| TEXAS INSTRUMENTS INCORPORATED
| Standard Linear and Logic Group
| IBIS Model of SN74LVCR162245
| 16-BIT BUS TRANSCEIVER WITH 3-STATE OUTPUTS
| This file contains package information for the following:
|  TSSOP 48-pin (DGG) package as [Component] LVCR162245_DGG
|  jrBGA 48-pin (GQL) package as [Component] LVCR162245_GQL
|  jrBGA 48-pin (ZQL) package as [Component] LVCR162245_ZQL
|  SSOP 48-pin (DL) package as [Component] LVCR162245_DL
| This device can be powered at the following Vccs:
|  2.5 volt Vcc
|  3.3 volt Vcc
| This file provides unique models under the [Model Selector] for each Vcc.
| For operation at a specific Vcc, select the appropriate model after each
| [Model Selector] keyword.
[IBIS Ver]   3.2
[Comment char]  |_char
[File Name]   sn74lvcr162245.ibs
[File Rev]   1.3 | a_die
[Date]   May 16, 2007
[Source]   Data created from TI-SPICE simulations at TI-SLL.
[Notes]   The following is an IBIS list for the SN74LVCR162245.
   Please contact sllibis@ti.com with questions and
   comments concerning SLL IBIS models.
   This IBIS model is created from a BA (back annotated netlist)
   - FILE REV HISTORY
   - 1.1 Release IBIS file on 12/20/04
   - 1.2 Release IBIS file on 5/8/07
   - 1.3 Release IBIS file on 7/20/07, using R_load of 50ohm
   - Non-monotonic data in pullup data due to damping resistor.
[Disclaimer] Property of Texas Instruments Incorporated.  Unauthorized
   reproduction and/or distribution is strictly prohibited.
   This product is protected under copyright law.
   Created  2007, (C) Copyright  2007, Texas Instruments
   Incorporated, All Rights Reserved
   UNLESS THERE IS A SIGNED, WRITTEN AGREEMENT TO THE
   CONTRARY, TEXAS INSTRUMENTS (TI) IS PROVIDING THE IBIS
   MODELS  AND WITHOUT ANY WARRANTY, EXPRESSED OR
   IMPLIED.  TI assumes no liability for:
   1) the accuracy of the IBIS models provided to your
   company;
   2) the proper functioning of these IBIS Models in your
   design or for any resulting applications; or
   3) infringement of patents, copyrights or intellectual
   property rights resulting from your use of these IBIS
   models.
   TI provides IBIS Models as a service to our customers.
   You and your company shall not distribute, sell or give
   these models to anyone else without prior written
   permission from TI.
   TI reserves the right to make changes to our products or
   to discontinue any semiconductor product or service
   without notice, and advises our customers to obtain the
   latest version of relevant information to verify, before
   placing orders, that the information being relied on is
   current.
   Please be aware that your receipt and use of the IBIS
   information provided shall serve as acceptance of these
   terms and conditions.  If you do not accept these terms,
   you should return or destroy the IBIS models and any
   other accompanying information immediately.
| Component SN74LVCR162245_DGG 48-PIN TSSOP
[Component]   SN74LVCR162245_DGG
[Manufacturer]   Texas Instruments, Inc.
[Package]
|   typ   min   max
R_pkg   6.200e-02   5.000e-02   7.800e-02
L_pkg   3.527e-09   3.128e-09   4.255e-09
C_pkg   5.300e-13   4.170e-13   6.850e-13
[Pin]   signal_name   model_name   R_pin   L_pin   C_pin
1   1DIR   LVCR162245_DIR   5.000e-02   4.250e-09   6.710e-13
2   1B1   LVCR162245_IO   5.700e-02   3.956e-09   6.740e-13
3   1B2   LVCR162245_IO   7.100e-02   3.922e-09   6.190e-13
4   GND   GND   7.800e-02   3.841e-09   6.180e-13
5   1B3   LVCR162245_IO   5.600e-02   3.535e-09   5.550e-13
6   1B4   LVCR162245_IO   5.800e-02   3.464e-09   5.030e-13
7   VCC   POWER   6.000e-02   3.362e-09   4.980e-13
8   1B5   LVCR162245_IO   6.100e-02   3.293e-09   4.620e-13
9   1B6   LVCR162245_IO   6.300e-02   3.240e-09   4.550e-13
10   GND   GND   6.300e-02   3.175e-09   4.420e-13
11   1B7   LVCR162245_IO   6.400e-02   3.153e-09   4.290e-13
12   1B8   LVCR162245_IO   6.500e-02   3.128e-09   4.180e-13
13   2B1   LVCR162245_IO   6.500e-02   3.128e-09   4.180e-13
14   2B2   LVCR162245_IO   6.400e-02   3.154e-09   4.290e-13
15   GND   GND   6.300e-02   3.174e-09   4.420e-13
16   2B3   LVCR162245_IO   6.300e-02   3.241e-09   4.550e-13
17   2B4   LVCR162245_IO   6.100e-02   3.293e-09   4.620e-13
18   VCC   POWER   6.000e-02   3.362e-09   4.970e-13
19   2B5   LVCR162245_IO   5.800e-02   3.464e-09   5.030e-13
20   2B6   LVCR162245_IO   5.600e-02   3.537e-09   5.600e-13
21   GND   GND   7.700e-02   3.839e-09   6.260e-13
22   2B7   LVCR162245_IO   7.100e-02   3.917e-09   6.270e-13
23   2B8   LVCR162245_IO   5.800e-02   3.955e-09   6.850e-13
24   2DIR   LVCR162245_DIR   5.200e-02   4.255e-09   6.790e-13
25   2NOE   LVCR162245_NOE   5.100e-02   4.254e-09   6.760e-13
26   2A8   LVCR162245_IO   5.800e-02   3.957e-09   6.790e-13
27   2A7   LVCR162245_IO   7.100e-02   3.920e-09   6.210e-13
28   GND   GND   7.800e-02   3.843e-09   6.220e-13
29   2A6   LVCR162245_IO   5.600e-02   3.539e-09   5.600e-13
30   2A5   LVCR162245_IO   5.800e-02   3.466e-09   5.030e-13
31   VCC   POWER   6.000e-02   3.363e-09   4.970e-13
32   2A4   LVCR162245_IO   6.100e-02   3.294e-09   4.620e-13
33   2A3   LVCR162245_IO   6.300e-02   3.241e-09   4.540e-13
34   GND   GND   6.300e-02   3.175e-09   4.410e-13
35   2A2   LVCR162245_IO   6.400e-02   3.153e-09   4.290e-13
36   2A1   LVCR162245_IO   6.500e-02   3.129e-09   4.170e-13
37   1A8   LVCR162245_IO   6.500e-02   3.129e-09   4.170e-13
38   1A7   LVCR162245_IO   6.400e-02   3.152e-09   4.290e-13
39   GND   GND   6.400e-02   3.176e-09   4.410e-13
40   1A6   LVCR162245_IO   6.300e-02   3.241e-09   4.540e-13
41   1A5   LVCR162245_IO   6.100e-02   3.293e-09   4.620e-13
42   VCC   POWER   6.000e-02   3.363e-09   4.970e-13
43   1A4   LVCR162245_IO   5.800e-02   3.464e-09   5.030e-13
44   1A3   LVCR162245_IO   5.600e-02   3.534e-09   5.610e-13
45   GND   GND   7.800e-02   3.841e-09   6.260e-13
46   1A2   LVCR162245_IO   7.100e-02   3.920e-09   6.220e-13
47   1A1   LVCR162245_IO   5.700e-02   3.955e-09   6.770e-13
48   1NOE   LVCR162245_NOE   5.100e-02   4.252e-09   6.720e-13
| Component SN74LVCR162245_GQL 48-PIN JRBGA
[Component]   SN74LVCR162245_GQL
[Manufacturer]   Texas Instruments, Inc.
[Package]
|   typ   min   max
R_pkg   7.900e-02   4.500e-02   9.400e-02
L_pkg   2.264e-09   1.398e-09   2.722e-09
C_pkg   3.060e-13   1.170e-13   4.040e-13
[Pin]   signal_name   model_name   R_pin   L_pin   C_pin
A1   1DIR   LVCR162245_DIR   5.100e-02   1.531e-09   2.100e-13
B3   GND   GND   9.400e-02   2.717e-09   3.830e-13
B2   1B1   LVCR162245_IO   7.300e-02   2.572e-09   3.120e-13
B1   1B2   LVCR162245_IO   7.100e-02   1.835e-09   2.320e-13
C3   VCC   POWER   9.400e-02   2.722e-09   3.920e-13
C2   1B3   LVCR162245_IO   8.900e-02   2.534e-09   3.500e-13
C1   1B4   LVCR162245_IO   7.100e-02   1.831e-09   2.310e-13
D2   1B5   LVCR162245_IO   9.000e-02   2.551e-09   3.520e-13
D3   GND   GND   9.400e-02   2.719e-09   4.030e-13
D1   1B6   LVCR162245_IO   7.200e-02   1.846e-09   2.440e-13
E2   1B7   LVCR162245_IO   8.900e-02   2.541e-09   3.510e-13
E1   1B8   LVCR162245_IO   7.200e-02   1.850e-09   2.270e-13
F1   2B1   LVCR162245_IO   7.200e-02   1.850e-09   2.270e-13
F2   2B2   LVCR162245_IO   8.900e-02   2.541e-09   3.510e-13
G1   2B3   LVCR162245_IO   7.200e-02   1.847e-09   2.440e-13
G3   GND   GND   9.300e-02   2.709e-09   3.820e-13
G2   2B4   LVCR162245_IO   9.000e-02   2.551e-09   3.520e-13
H1   2B5   LVCR162245_IO   7.000e-02   1.830e-09   2.310e-13
H2   2B6   LVCR162245_IO   8.800e-02   2.524e-09   3.500e-13
H3   VCC   POWER   9.400e-02   2.721e-09   3.920e-13
J1   2B7   LVCR162245_IO   7.100e-02   1.851e-09   2.330e-13
J2   2B8   LVCR162245_IO   5.600e-02   2.605e-09   3.900e-13
J3   GND   GND   9.300e-02   2.709e-09   3.820e-13
K1   2DIR   LVCR162245_DIR   4.500e-02   1.398e-09   1.170e-13
K6   2NOE   LVCR162245_NOE   4.500e-02   1.512e-09   1.930e-13
J4   GND   GND   9.300e-02   2.703e-09   3.820e-13
J5   2A8   LVCR162245_IO   5.500e-02   2.492e-09   3.130e-13
J6   2A7   LVCR162245_IO   7.000e-02   1.821e-09   2.300e-13
H4   VCC   POWER   9.400e-02   2.722e-09   3.910e-13
H5   2A6   LVCR162245_IO   8.900e-02   2.529e-09   3.500e-13
H6   2A5   LVCR162245_IO   7.100e-02   1.826e-09   2.300e-13
G5   2A4   LVCR162245_IO   9.000e-02   2.551e-09   3.520e-13
G4   GND   GND   9.400e-02   2.719e-09   4.040e-13
G6   2A3   LVCR162245_IO   7.200e-02   1.846e-09   2.440e-13
F5   2A2   LVCR162245_IO   8.800e-02   2.510e-09   3.490e-13
F6   2A1   LVCR162245_IO   7.200e-02   1.850e-09   2.270e-13
E6   1A8   LVCR162245_IO   7.100e-02   1.850e-09   2.270e-13
E5   1A7   LVCR162245_IO   8.900e-02   2.529e-09   3.500e-13
D6   1A6   LVCR162245_IO   7.200e-02   1.847e-09   2.430e-13
D4   GND   GND   9.300e-02   2.705e-09   3.820e-13
D5   1A5   LVCR162245_IO   8.900e-02   2.550e-09   3.520e-13
C6   1A4   LVCR162245_IO   7.100e-02   1.827e-09   2.300e-13
C5   1A3   LVCR162245_IO   8.900e-02   2.539e-09   3.500e-13
C4   VCC   POWER   9.400e-02   2.722e-09   3.910e-13
B6   1A2   LVCR162245_IO   7.100e-02   1.831e-09   2.270e-13
B5   1A1   LVCR162245_IO   7.300e-02   2.685e-09   3.800e-13
A6   1NOE   LVCR162245_NOE   5.100e-02   1.417e-09   1.330e-13
| Component SN74LVCR162245_ZQL 48-PIN JRBGA
[Component]   SN74LVCR162245_ZQL
[Manufacturer]   Texas Instruments, Inc.
[Package]
|   typ   min   max
R_pkg   7.900e-02   4.500e-02   9.400e-02
L_pkg   2.264e-09   1.398e-09   2.722e-09
C_pkg   3.060e-13   1.170e-13   4.040e-13
[Pin]   signal_name   model_name   R_pin   L_pin   C_pin
A1   1DIR   LVCR162245_DIR   5.100e-02   1.531e-09   2.100e-13
B3   GND   GND   9.400e-02   2.717e-09   3.830e-13
B2   1B1   LVCR162245_IO   7.300e-02   2.572e-09   3.120e-13
B1   1B2   LVCR162245_IO   7.100e-02   1.835e-09   2.320e-13
C3   VCC   POWER   9.400e-02   2.722e-09   3.920e-13
C2   1B3   LVCR162245_IO   8.900e-02   2.534e-09   3.500e-13
C1   1B4   LVCR162245_IO   7.100e-02   1.831e-09   2.310e-13
D2   1B5   LVCR162245_IO   9.000e-02   2.551e-09   3.520e-13
D3   GND   GND   9.400e-02   2.719e-09   4.030e-13
D1   1B6   LVCR162245_IO   7.200e-02   1.846e-09   2.440e-13
E2   1B7   LVCR162245_IO   8.900e-02   2.541e-09   3.510e-13
E1   1B8   LVCR162245_IO   7.200e-02   1.850e-09   2.270e-13
F1   2B1   LVCR162245_IO   7.200e-02   1.850e-09   2.270e-13
F2   2B2   LVCR162245_IO   8.900e-02   2.541e-09   3.510e-13
G1   2B3   LVCR162245_IO   7.200e-02   1.847e-09   2.440e-13
G3   GND   GND   9.300e-02   2.709e-09   3.820e-13
G2   2B4   LVCR162245_IO   9.000e-02   2.551e-09   3.520e-13
H1   2B5   LVCR162245_IO   7.000e-02   1.830e-09   2.310e-13
H2   2B6   LVCR162245_IO   8.800e-02   2.524e-09   3.500e-13
H3   VCC   POWER   9.400e-02   2.721e-09   3.920e-13
J1   2B7   LVCR162245_IO   7.100e-02   1.851e-09   2.330e-13
J2   2B8   LVCR162245_IO   5.600e-02   2.605e-09   3.900e-13
J3   GND   GND   9.300e-02   2.709e-09   3.820e-13
K1   2DIR   LVCR162245_DIR   4.500e-02   1.398e-09   1.170e-13
K6   2NOE   LVCR162245_NOE   4.500e-02   1.512e-09   1.930e-13
J4   GND   GND   9.300e-02   2.703e-09   3.820e-13
J5   2A8   LVCR162245_IO   5.500e-02   2.492e-09   3.130e-13
J6   2A7   LVCR162245_IO   7.000e-02   1.821e-09   2.300e-13
H4   VCC   POWER   9.400e-02   2.722e-09   3.910e-13
H5   2A6   LVCR162245_IO   8.900e-02   2.529e-09   3.500e-13
H6   2A5   LVCR162245_IO   7.100e-02   1.826e-09   2.300e-13
G5   2A4   LVCR162245_IO   9.000e-02   2.551e-09   3.520e-13
G4   GND   GND   9.400e-02   2.719e-09   4.040e-13
G6   2A3   LVCR162245_IO   7.200e-02   1.846e-09   2.440e-13
F5   2A2   LVCR162245_IO   8.800e-02   2.510e-09   3.490e-13
F6   2A1   LVCR162245_IO   7.200e-02   1.850e-09   2.270e-13
E6   1A8   LVCR162245_IO   7.100e-02   1.850e-09   2.270e-13
E5   1A7   LVCR162245_IO   8.900e-02   2.529e-09   3.500e-13
D6   1A6   LVCR162245_IO   7.200e-02   1.847e-09   2.430e-13
D4   GND   GND   9.300e-02   2.705e-09   3.820e-13
D5   1A5   LVCR162245_IO   8.900e-02   2.550e-09   3.520e-13
C6   1A4   LVCR162245_IO   7.100e-02   1.827e-09   2.300e-13
C5   1A3   LVCR162245_IO   8.900e-02   2.539e-09   3.500e-13
C4   VCC   POWER   9.400e-02   2.722e-09   3.910e-13
B6   1A2   LVCR162245_IO   7.100e-02   1.831e-09   2.270e-13
B5   1A1   LVCR162245_IO   7.300e-02   2.685e-09   3.800e-13
A6   1NOE   LVCR162245_NOE   5.100e-02   1.417e-09   1.330e-13
| Component SN74LVCR162245_DL 48-PIN SSOP
[Component]   SN74LVCR162245_DL
[Manufacturer]   Texas Instruments, Inc.
[Package]
|   typ   min   max
R_pkg   4.800e-02   3.800e-02   5.300e-02
L_pkg   6.046e-09   5.084e-09   7.968e-09
C_pkg   8.130e-13   5.690e-13   1.157e-12
[Pin]   signal_name   model_name   R_pin   L_pin   C_pin
1   1DIR   LVCR162245_DIR   4.600e-02   7.968e-09   1.017e-12
2   1B1   LVCR162245_IO   4.400e-02   7.299e-09   1.157e-12
3   1B2   LVCR162245_IO   4.300e-02   6.765e-09   1.058e-12
4   GND   GND   4.100e-02   6.269e-09   9.330e-13
5   1B3   LVCR162245_IO   3.800e-02   5.856e-09   8.290e-13
6   1B4   LVCR162245_IO   4.600e-02   5.802e-09   7.900e-13
7   VCC   POWER   5.000e-02   5.656e-09   7.380e-13
8   1B5   LVCR162245_IO   5.300e-02   5.500e-09   6.430e-13
9   1B6   LVCR162245_IO   5.200e-02   5.304e-09   6.060e-13
10   GND   GND   5.300e-02   5.189e-09   5.830e-13
11   1B7   LVCR162245_IO   5.100e-02   5.084e-09   5.690e-13
12   1B8   LVCR162245_IO   5.300e-02   5.862e-09   8.330e-13
13   2B1   LVCR162245_IO   5.300e-02   5.862e-09   8.330e-13
14   2B2   LVCR162245_IO   5.100e-02   5.084e-09   5.690e-13
15   GND   GND   5.300e-02   5.189e-09   5.830e-13
16   2B3   LVCR162245_IO   5.200e-02   5.304e-09   6.060e-13
17   2B4   LVCR162245_IO   5.300e-02   5.500e-09   6.430e-13
18   VCC   POWER   5.000e-02   5.656e-09   7.380e-13
19   2B5   LVCR162245_IO   4.600e-02   5.802e-09   7.900e-13
20   2B6   LVCR162245_IO   3.800e-02   5.856e-09   8.290e-13
21   GND   GND   4.100e-02   6.269e-09   9.330e-13
22   2B7   LVCR162245_IO   4.300e-02   6.765e-09   1.058e-12
23   2B8   LVCR162245_IO   4.400e-02   7.299e-09   1.157e-12
24   2DIR   LVCR162245_DIR   4.600e-02   7.968e-09   1.017e-12
25   2NOE   LVCR162245_NOE   4.600e-02   7.968e-09   1.017e-12
26   2A8   LVCR162245_IO   4.400e-02   7.299e-09   1.157e-12
27   2A7   LVCR162245_IO   4.300e-02   6.765e-09   1.058e-12
28   GND   GND   4.100e-02   6.269e-09   9.330e-13
29   2A6   LVCR162245_IO   3.800e-02   5.856e-09   8.290e-13
30   2A5   LVCR162245_IO   4.600e-02   5.802e-09   7.900e-13
31   VCC   POWER   5.000e-02   5.656e-09   7.380e-13
32   2A4   LVCR162245_IO   5.300e-02   5.500e-09   6.430e-13
33   2A3   LVCR162245_IO   5.200e-02   5.304e-09   6.060e-13
34   GND   GND   5.300e-02   5.189e-09   5.830e-13
35   2A2   LVCR162245_IO   5.100e-02   5.084e-09   5.690e-13
36   2A1   LVCR162245_IO   5.300e-02   5.862e-09   8.330e-13
37   1A8   LVCR162245_IO   5.300e-02   5.862e-09   8.330e-13
38   1A7   LVCR162245_IO   5.100e-02   5.084e-09   5.690e-13
39   GND   GND   5.300e-02   5.189e-09   5.830e-13
40   1A6   LVCR162245_IO   5.200e-02   5.304e-09   6.060e-13
41   1A5   LVCR162245_IO   5.300e-02   5.500e-09   6.430e-13
42   VCC   POWER   5.000e-02   5.656e-09   7.380e-13
43   1A4   LVCR162245_IO   4.600e-02   5.802e-09   7.900e-13
44   1A3   LVCR162245_IO   3.800e-02   5.856e-09   8.290e-13
45   GND   GND   4.100e-02   6.269e-09   9.330e-13
46   1A2   LVCR162245_IO   4.300e-02   6.765e-09   1.058e-12
47   1A1   LVCR162245_IO   4.400e-02   7.299e-09   1.157e-12
48   1NOE   LVCR162245_NOE   4.600e-02   7.967e-09   1.017e-12
| Model LVCR162245_NOE
[Model Selector]   LVCR162245_NOE
LVCR162245_NOE_25   2.5 volt Vcc
LVCR162245_NOE_33   3.3 volt Vcc
| Model LVCR162245_DIR
[Model Selector]   LVCR162245_DIR
LVCR162245_DIR_25   2.5 volt Vcc
LVCR162245_DIR_33   3.3 volt Vcc
| Model LVCR162245_IO
[Model Selector]   LVCR162245_IO
LVCR162245_IO_25   2.5 volt Vcc
LVCR162245_IO_33   3.3 volt Vcc
| Models and submodels in the file (6): LVCR162245_NOE_25 (Input), LVCR162245_NOE_33 (Input), LVCR162245_DIR_25 (Input), LVCR162245_DIR_33 (Input), LVCR162245_IO_25 (I/O), LVCR162245_IO_33 (I/O)
